| TEXAS INSTRUMENTS INCORPORATED
| Standard Linear and Logic Group
| IBIS Model of SN74LVC16244A
| 16-BIT BUFFER/DRIVER WITH 3-STATE OUTPUTS
| This file contains package information for the following:
|  TSSOP 48-pin (DGG) package as [Component] LVC16244A_DGG
|  SSOP 48-pin (DL) package as [Component] LVC16244A_DL
|  TVSOP 48-pin (DGV) package as [Component] LVC16244A_DGV
|  VFBGA 48-pin (GQL) package as [Component] LVC16244A_GQL
| This device can be powered at the following Vccs:
|  3.3 volt Vcc
|  2.5 volt Vcc
|  1.8 volt Vcc
| This file provides unique models under the [Model Selector] for each Vcc.
| For operation at a specific Vcc, select the appropriate model after each
| [Model Selector] keyword.
[IBIS Ver]   3.2
[Comment char]  |_char
[File Name]   sn74lvc16244a.ibs
[File Rev]   1.1 | e_die
[Date]   March 26, 2002
[Source]   Data created from TI-SPICE simulations at TI-SLL.
[Notes]   The following is an IBIS list for the LVC16244A.
   Please contact sllibis@ti.com with questions and
   comments concerning SLL IBIS models.
   -As there is no power clamp diode in the Input and Output
   Models, we removed the Pwr Clamp table data from those
   Models.
   -Due to the fact that the Device is 5-V Input/Output
   tolarent, the pullup data has some Non-Monotonic Warnings.
   -C_comp values are taken at a different test condition than
   the data sheet.
[Disclaimer] Property of Texas Instruments Incorporated.  Unauthorized
   reproduction and/or distribution is strictly prohibited.
   This product is protected under copyright law.
   Created  2002, (C) Copyright  2002, Texas Instruments
   Incorporated, All Rights Reserved
   UNLESS THERE IS A SIGNED, WRITTEN AGREEMENT TO THE
   CONTRARY, TEXAS INSTRUMENTS (TI) IS PROVIDING THE IBIS
   MODELS  AND WITHOUT ANY WARRANTY, EXPRESSED OR
   IMPLIED.  TI assumes no liability for:
   1) the accuracy of the IBIS models provided to your
   company;
   2) the proper functioning of these IBIS Models in your
   design or for any resulting applications; or
   3) infringement of patents, copyrights or intellectual
   property rights resulting from your use of these IBIS
   models.
   TI provides IBIS Models as a service to our customers.
   You and your company shall not distribute, sell or give
   these models to anyone else without prior written
   permission from TI.
   TI reserves the right to make changes to our products or
   to discontinue any semiconductor product or service
   without notice, and advises our customers to obtain the
   latest version of relevant information to verify, before
   placing orders, that the information being relied on is
   current.
   Please be aware that your receipt and use of the IBIS
   information provided shall serve as acceptance of these
   terms and conditions.  If you do not accept these terms,
   you should return or destroy the IBIS models and any
   other accompanying information immediately.
| Component LVC16244A_DGG 48-pin TSSOP
[Component]   LVC16244A_DGG
[Manufacturer]   Texas Instruments, Inc.
[Package]
|   typ   min   max
R_pkg   4.400e-02   3.800e-02   5.100e-02
L_pkg   3.019e-09   2.486e-09   4.099e-09
C_pkg   5.070e-13   3.340e-13   8.090e-13
[Pin]   signal_name   model_name   R_pin   L_pin   C_pin
1   1NOE   LVC16244A_OEIN   4.100e-02   4.017e-09   7.590e-13
2   1Y1   LVC16244A_OUT   4.200e-02   3.737e-09   7.920e-13
3   1Y2   LVC16244A_OUT   4.200e-02   3.480e-09   6.610e-13
4   GND   GND   3.800e-02   3.131e-09   5.750e-13
5   1Y3   LVC16244A_OUT   4.700e-02   3.122e-09   5.660e-13
6   1Y4   LVC16244A_OUT   4.300e-02   2.948e-09   5.040e-13
7   VCC   POWER   4.500e-02   2.845e-09   3.970e-13
8   2Y1   LVC16244A_OUT   4.900e-02   2.835e-09   3.940e-13
9   2Y2   LVC16244A_OUT   4.800e-02   2.715e-09   3.780e-13
10   GND   GND   5.000e-02   2.664e-09   3.630e-13
11   2Y3   LVC16244A_OUT   5.000e-02   2.585e-09   3.480e-13
12   2Y4   LVC16244A_OUT   4.900e-02   2.550e-09   3.370e-13
13   3Y1   LVC16244A_OUT   4.900e-02   2.541e-09   3.360e-13
14   3Y2   LVC16244A_OUT   5.000e-02   2.574e-09   3.480e-13
15   GND   GND   4.900e-02   2.618e-09   3.590e-13
16   3Y3   LVC16244A_OUT   4.600e-02   2.671e-09   3.750e-13
17   3Y4   LVC16244A_OUT   4.500e-02   2.754e-09   3.890e-13
18   VCC   POWER   4.400e-02   2.823e-09   4.500e-13
19   4Y1   LVC16244A_OUT   4.200e-02   2.968e-09   5.030e-13
20   4Y2   LVC16244A_OUT   5.100e-02   3.108e-09   5.350e-13
21   GND   GND   4.200e-02   3.175e-09   5.870e-13
22   4Y3   LVC16244A_OUT   4.100e-02   3.449e-09   6.780e-13
23   4Y4   LVC16244A_OUT   4.400e-02   3.766e-09   8.040e-13
24   4NOE   LVC16244A_OEIN   4.300e-02   4.065e-09   7.610e-13
25   3NOE   LVC16244A_OEIN   4.100e-02   3.994e-09   7.570e-13
26   4A4   LVC16244A_IN   3.900e-02   3.649e-09   7.890e-13
27   4A3   LVC16244A_IN   3.800e-02   3.362e-09   6.600e-13
28   GND   GND   3.800e-02   3.082e-09   5.740e-13
29   4A2   LVC16244A_IN   4.400e-02   2.990e-09   5.220e-13
30   4A1   LVC16244A_IN   4.100e-02   2.917e-09   4.950e-13
31   VCC   POWER   4.300e-02   2.820e-09   4.480e-13
32   3A4   LVC16244A_IN   4.300e-02   2.699e-09   3.850e-13
33   3A3   LVC16244A_IN   4.500e-02   2.628e-09   3.720e-13
34   GND   GND   4.600e-02   2.556e-09   3.560e-13
35   3A2   LVC16244A_IN   4.600e-02   2.495e-09   3.440e-13
36   3A1   LVC16244A_IN   4.700e-02   2.487e-09   3.340e-13
37   2A4   LVC16244A_IN   4.700e-02   2.490e-09   3.350e-13
38   2A3   LVC16244A_IN   4.600e-02   2.486e-09   3.430e-13
39   GND   GND   4.500e-02   2.566e-09   3.560e-13
40   2A2   LVC16244A_IN   4.400e-02   2.639e-09   3.740e-13
41   2A1   LVC16244A_IN   4.300e-02   2.701e-09   3.860e-13
42   VCC   POWER   4.300e-02   2.817e-09   4.500e-13
43   1A4   LVC16244A_IN   4.100e-02   2.935e-09   5.010e-13
44   1A3   LVC16244A_IN   4.700e-02   3.035e-09   5.290e-13
45   GND   GND   4.300e-02   3.171e-09   5.890e-13
46   1A2   LVC16244A_IN   4.000e-02   3.415e-09   6.820e-13
47   1A1   LVC16244A_IN   4.300e-02   3.741e-09   8.090e-13
48   2NOE   LVC16244A_OEIN   4.400e-02   4.099e-09   7.640e-13
| Component LVC16244A_DL 48-pin SSOP
[Component]   LVC16244A_DL
[Manufacturer]   Texas Instruments, Inc.
[Package]
|   typ   min   max
R_pkg   4.800e-02   3.800e-02   5.300e-02
L_pkg   6.046e-09   5.084e-09   7.968e-09
C_pkg   8.130e-13   5.690e-13   1.157e-12
[Pin]   signal_name   model_name   R_pin   L_pin   C_pin
1   1NOE   LVC16244A_OEIN   4.600e-02   7.968e-09   1.017e-12
2   1Y1   LVC16244A_OUT   4.400e-02   7.299e-09   1.157e-12
3   1Y2   LVC16244A_OUT   4.300e-02   6.765e-09   1.058e-12
4   GND   GND   4.100e-02   6.269e-09   9.330e-13
5   1Y3   LVC16244A_OUT   3.800e-02   5.856e-09   8.290e-13
6   1Y4   LVC16244A_OUT   4.600e-02   5.802e-09   7.900e-13
7   VCC   POWER   5.000e-02   5.656e-09   7.380e-13
8   2Y1   LVC16244A_OUT   5.300e-02   5.500e-09   6.430e-13
9   2Y2   LVC16244A_OUT   5.200e-02   5.304e-09   6.060e-13
10   GND   GND   5.300e-02   5.189e-09   5.830e-13
11   2Y3   LVC16244A_OUT   5.100e-02   5.084e-09   5.690e-13
12   2Y4   LVC16244A_OUT   5.300e-02   5.862e-09   8.330e-13
13   3Y1   LVC16244A_OUT   5.300e-02   5.862e-09   8.330e-13
14   3Y2   LVC16244A_OUT   5.100e-02   5.084e-09   5.690e-13
15   GND   GND   5.300e-02   5.189e-09   5.830e-13
16   3Y3   LVC16244A_OUT   5.200e-02   5.304e-09   6.060e-13
17   3Y4   LVC16244A_OUT   5.300e-02   5.500e-09   6.430e-13
18   VCC   POWER   5.000e-02   5.656e-09   7.380e-13
19   4Y1   LVC16244A_OUT   4.600e-02   5.802e-09   7.900e-13
20   4Y2   LVC16244A_OUT   3.800e-02   5.856e-09   8.290e-13
21   GND   GND   4.100e-02   6.269e-09   9.330e-13
22   4Y3   LVC16244A_OUT   4.300e-02   6.765e-09   1.058e-12
23   4Y4   LVC16244A_OUT   4.400e-02   7.299e-09   1.157e-12
24   4NOE   LVC16244A_OEIN   4.600e-02   7.968e-09   1.017e-12
25   3NOE   LVC16244A_OEIN   4.600e-02   7.968e-09   1.017e-12
26   4A4   LVC16244A_IN   4.400e-02   7.299e-09   1.157e-12
27   4A3   LVC16244A_IN   4.300e-02   6.765e-09   1.058e-12
28   GND   GND   4.100e-02   6.269e-09   9.330e-13
29   4A2   LVC16244A_IN   3.800e-02   5.856e-09   8.290e-13
30   4A1   LVC16244A_IN   4.600e-02   5.802e-09   7.900e-13
31   VCC   POWER   5.000e-02   5.656e-09   7.380e-13
32   3A4   LVC16244A_IN   5.300e-02   5.500e-09   6.430e-13
33   3A3   LVC16244A_IN   5.200e-02   5.304e-09   6.060e-13
34   GND   GND   5.300e-02   5.189e-09   5.830e-13
35   3A2   LVC16244A_IN   5.100e-02   5.084e-09   5.690e-13
36   3A1   LVC16244A_IN   5.300e-02   5.862e-09   8.330e-13
37   2A4   LVC16244A_IN   5.300e-02   5.862e-09   8.330e-13
38   2A3   LVC16244A_IN   5.100e-02   5.084e-09   5.690e-13
39   GND   GND   5.300e-02   5.189e-09   5.830e-13
40   2A2   LVC16244A_IN   5.200e-02   5.304e-09   6.060e-13
41   2A1   LVC16244A_IN   5.300e-02   5.500e-09   6.430e-13
42   VCC   POWER   5.000e-02   5.656e-09   7.380e-13
43   1A4   LVC16244A_IN   4.600e-02   5.802e-09   7.900e-13
44   1A3   LVC16244A_IN   3.800e-02   5.856e-09   8.290e-13
45   GND   GND   4.100e-02   6.269e-09   9.330e-13
46   1A2   LVC16244A_IN   4.300e-02   6.765e-09   1.058e-12
47   1A1   LVC16244A_IN   4.400e-02   7.299e-09   1.157e-12
48   2NOE   LVC16244A_OEIN   4.600e-02   7.967e-09   1.017e-12
| Component LVC16244A_DGV 48-pin TVSOP
[Component]   LVC16244A_DGV
[Manufacturer]   Texas Instruments, Inc.
[Package]
|   typ   min   max
R_pkg   7.000e-02   4.900e-02   8.500e-02
L_pkg   3.013e-09   2.743e-09   3.408e-09
C_pkg   3.710e-13   2.940e-13   5.110e-13
[Pin]   signal_name   model_name   R_pin   L_pin   C_pin
1   1NOE   LVC16244A_OEIN   4.900e-02   3.393e-09   4.970e-13
2   1Y1   LVC16244A_OUT   6.000e-02   3.250e-09   5.020e-13
3   1Y2   LVC16244A_OUT   7.700e-02   3.310e-09   4.510e-13
4   GND   GND   8.500e-02   3.299e-09   4.040e-13
5   1Y3   LVC16244A_OUT   8.300e-02   3.136e-09   3.600e-13
6   1Y4   LVC16244A_OUT   7.700e-02   3.019e-09   3.630e-13
7   VCC   POWER   6.500e-02   2.882e-09   3.490e-13
8   2Y1   LVC16244A_OUT   6.600e-02   2.829e-09   3.140e-13
9   2Y2   LVC16244A_OUT   6.700e-02   2.796e-09   3.140e-13
10   GND   GND   6.900e-02   2.754e-09   3.080e-13
11   2Y3   LVC16244A_OUT   7.000e-02   2.753e-09   3.010e-13
12   2Y4   LVC16244A_OUT   7.100e-02   2.745e-09   2.940e-13
13   3Y1   LVC16244A_OUT   7.000e-02   2.744e-09   2.940e-13
14   3Y2   LVC16244A_OUT   7.000e-02   2.754e-09   3.010e-13
15   GND   GND   6.900e-02   2.754e-09   3.080e-13
16   3Y3   LVC16244A_OUT   6.700e-02   2.796e-09   3.140e-13
17   3Y4   LVC16244A_OUT   6.600e-02   2.829e-09   3.140e-13
18   VCC   POWER   6.500e-02   2.883e-09   3.500e-13
19   4Y1   LVC16244A_OUT   7.500e-02   3.014e-09   3.630e-13
20   4Y2   LVC16244A_OUT   8.000e-02   3.128e-09   3.580e-13
21   GND   GND   8.400e-02   3.295e-09   4.030e-13
22   4Y3   LVC16244A_OUT   7.800e-02   3.311e-09   4.520e-13
23   4Y4   LVC16244A_OUT   6.200e-02   3.259e-09   5.010e-13
24   4NOE   LVC16244A_OEIN   5.200e-02   3.404e-09   4.960e-13
25   3NOE   LVC16244A_OEIN   5.300e-02   3.397e-09   5.050e-13
26   4A4   LVC16244A_IN   6.200e-02   3.249e-09   5.110e-13
27   4A3   LVC16244A_IN   7.700e-02   3.308e-09   4.530e-13
28   GND   GND   8.200e-02   3.289e-09   4.030e-13
29   4A2   LVC16244A_IN   7.800e-02   3.121e-09   3.590e-13
30   4A1   LVC16244A_IN   7.400e-02   3.010e-09   3.630e-13
31   VCC   POWER   6.500e-02   2.883e-09   3.490e-13
32   3A4   LVC16244A_IN   6.700e-02   2.829e-09   3.140e-13
33   3A3   LVC16244A_IN   6.700e-02   2.795e-09   3.140e-13
34   GND   GND   6.900e-02   2.753e-09   3.070e-13
35   3A2   LVC16244A_IN   7.000e-02   2.753e-09   3.010e-13
36   3A1   LVC16244A_IN   7.000e-02   2.743e-09   2.940e-13
37   2A4   LVC16244A_IN   7.000e-02   2.743e-09   2.940e-13
38   2A3   LVC16244A_IN   7.000e-02   2.753e-09   3.010e-13
39   GND   GND   6.900e-02   2.754e-09   3.070e-13
40   2A2   LVC16244A_IN   6.800e-02   2.797e-09   3.140e-13
41   2A1   LVC16244A_IN   6.700e-02   2.830e-09   3.140e-13
42   VCC   POWER   6.400e-02   2.880e-09   3.490e-13
43   1A4   LVC16244A_IN   7.200e-02   3.004e-09   3.620e-13
44   1A3   LVC16244A_IN   7.800e-02   3.121e-09   3.590e-13
45   GND   GND   8.400e-02   3.296e-09   4.030e-13
46   1A2   LVC16244A_IN   7.700e-02   3.308e-09   4.510e-13
47   1A1   LVC16244A_IN   6.200e-02   3.258e-09   4.990e-13
48   2NOE   LVC16244A_OEIN   5.300e-02   3.408e-09   4.940e-13
| Component LVC16244A_GQL 48-pin VFBGA
[Component]   LVC16244A_GQL
[Manufacturer]   Texas Instruments, Inc.
[Package]
|   typ   min   max
R_pkg   7.900e-02   4.500e-02   9.400e-02
L_pkg   2.264e-09   1.398e-09   2.722e-09
C_pkg   3.060e-13   1.170e-13   4.040e-13
[Pin]   signal_name   model_name   R_pin   L_pin   C_pin
A1   1NOE   LVC16244A_OEIN   5.100e-02   1.531e-09   2.100e-13
B2   1Y1   LVC16244A_OUT   7.300e-02   2.572e-09   3.120e-13
B1   1Y2   LVC16244A_OUT   7.100e-02   1.835e-09   2.320e-13
B3   GND   GND   9.400e-02   2.717e-09   3.830e-13
C2   1Y3   LVC16244A_OUT   8.900e-02   2.534e-09   3.500e-13
C1   1Y4   LVC16244A_OUT   7.100e-02   1.831e-09   2.310e-13
C3   VCC   POWER   9.400e-02   2.722e-09   3.920e-13
D2   2Y1   LVC16244A_OUT   9.000e-02   2.551e-09   3.520e-13
D1   2Y2   LVC16244A_OUT   7.200e-02   1.846e-09   2.440e-13
D3   GND   GND   9.400e-02   2.719e-09   4.030e-13
E2   2Y3   LVC16244A_OUT   8.900e-02   2.541e-09   3.510e-13
E1   2Y4   LVC16244A_OUT   7.200e-02   1.850e-09   2.270e-13
F1   3Y1   LVC16244A_OUT   7.200e-02   1.850e-09   2.270e-13
F2   3Y2   LVC16244A_OUT   8.900e-02   2.541e-09   3.510e-13
G3   GND   GND   9.400e-02   2.718e-09   4.040e-13
G1   3Y3   LVC16244A_OUT   7.200e-02   1.847e-09   2.440e-13
G2   3Y4   LVC16244A_OUT   9.000e-02   2.551e-09   3.520e-13
H3   VCC   POWER   9.400e-02   2.721e-09   3.920e-13
H1   4Y1   LVC16244A_OUT   7.000e-02   1.830e-09   2.310e-13
H2   4Y2   LVC16244A_OUT   8.800e-02   2.524e-09   3.500e-13
J3   GND   GND   9.300e-02   2.709e-09   3.820e-13
J1   4Y3   LVC16244A_OUT   7.100e-02   1.851e-09   2.330e-13
J2   4Y4   LVC16244A_OUT   5.600e-02   2.605e-09   3.900e-13
K1   4NOE   LVC16244A_OEIN   4.500e-02   1.398e-09   1.170e-13
K6   3NOE   LVC16244A_OEIN   4.500e-02   1.512e-09   1.930e-13
J5   4A4   LVC16244A_IN   5.500e-02   2.492e-09   3.130e-13
J6   4A3   LVC16244A_IN   7.000e-02   1.821e-09   2.300e-13
J4   GND   GND   9.300e-02   2.703e-09   3.820e-13
H5   4A2   LVC16244A_IN   8.900e-02   2.529e-09   3.500e-13
H6   4A1   LVC16244A_IN   7.100e-02   1.826e-09   2.300e-13
H4   VCC   POWER   9.400e-02   2.722e-09   3.910e-13
G5   3A4   LVC16244A_IN   9.000e-02   2.551e-09   3.520e-13
G6   3A3   LVC16244A_IN   7.200e-02   1.846e-09   2.440e-13
G4   GND   GND   9.400e-02   2.719e-09   4.040e-13
F5   3A2   LVC16244A_IN   8.800e-02   2.510e-09   3.490e-13
F6   3A1   LVC16244A_IN   7.200e-02   1.850e-09   2.270e-13
E6   2A4   LVC16244A_IN   7.100e-02   1.850e-09   2.270e-13
E5   2A3   LVC16244A_IN   8.900e-02   2.529e-09   3.500e-13
D4   GND   GND   9.400e-02   2.719e-09   4.030e-13
D6   2A2   LVC16244A_IN   7.200e-02   1.847e-09   2.430e-13
D5   2A1   LVC16244A_IN   8.900e-02   2.550e-09   3.520e-13
C4   VCC   POWER   9.400e-02   2.722e-09   3.910e-13
C6   1A4   LVC16244A_IN   7.100e-02   1.827e-09   2.300e-13
C5   1A3   LVC16244A_IN   8.900e-02   2.539e-09   3.500e-13
B4   GND   GND   9.300e-02   2.705e-09   3.820e-13
B6   1A2   LVC16244A_IN   7.100e-02   1.831e-09   2.270e-13
B5   1A1   LVC16244A_IN   7.300e-02   2.685e-09   3.800e-13
A6   2NOE   LVC16244A_OEIN   5.100e-02   1.417e-09   1.330e-13
| Model LVC16244A_IN
[Model Selector]   LVC16244A_IN
LVC16244A_IN_33   3.3 volt Vcc
LVC16244A_IN_25   2.5 volt Vcc
LVC16244A_IN_18   1.8 volt Vcc
| Model LVC16244A_OEIN
[Model Selector]   LVC16244A_OEIN
LVC16244A_OEIN_33   3.3 volt Vcc
LVC16244A_OEIN_25   2.5 volt Vcc
LVC16244A_OEIN_18   1.8 volt Vcc
| Model LVC16244A_OUT
[Model Selector]   LVC16244A_OUT
LVC16244A_OUT_33   3.3 volt Vcc
LVC16244A_OUT_25   2.5 volt Vcc
LVC16244A_OUT_18   1.8 volt Vcc
| Models and submodels in the file (9): LVC16244A_IN_33 (Input), LVC16244A_IN_25 (Input), LVC16244A_IN_18 (Input), LVC16244A_OEIN_33 (Input), LVC16244A_OEIN_25 (Input), LVC16244A_OEIN_18 (Input), LVC16244A_OUT_33 (3-state), LVC16244A_OUT_25 (3-state), LVC16244A_OUT_18 (3-state)
